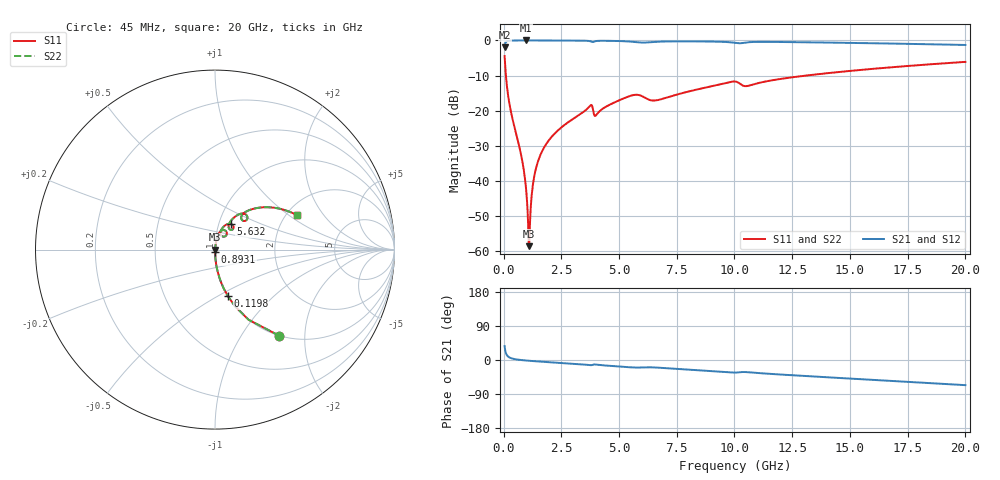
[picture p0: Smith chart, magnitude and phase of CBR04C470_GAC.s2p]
! S-parameter model data by Modelithics Inc.  support@modelithics.com 813-866-6335  Tampa FL USA
! S-Parameter data specifications:
! Substrate: 20-mil Rogers 4350B, substrate thickness, H=0.508mm, Dielectric constant, Er=3.75
! PCB Mounting Pad Footprint: Pad width, PadW=0.52mm , Pad length, PadL=0.52mm , Pad gap, PadG (edge-to-edge)=0.28mm , Reference planes=1.32mm apart
#  GHz  S  MA  R 50
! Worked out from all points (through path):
!   801 points, 45 MHz to 20 GHz, reference 50 ohm
!   highest |S21| = -0.01 dB at 967.9 MHz (marker M1); lowest = -1.9 dB at 45 MHz (marker M2)
!   group delay of S21, straight-line fit = 9.44 ps
!   lowest |S11| = -58.6 dB at 1.093 GHz (marker M3), VSWR 1.00, Z = 50.1 - j0.0592 ohm
!   |S11| at or under -10 dB: 100.8 MHz to 13.11 GHz (13.01 GHz wide, 197 % of centre)
!   |S22| runs from -58.6 to -4.4 dB; largest |S21 - S12| = 0
!   S11 on the Smith chart (normalised r, x): 45 MHz: 1.00, -1.50; 119.8 MHz: 1.00, -0.56; 893.1 MHz: 1.00, -0.03; 5.632 GHz: 1.14, +0.33; 20 GHz: 2.27, +1.16
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0.045  0.5995 -53.2  0.8002 36.8  0.8002 36.8  0.5995 -53.2
0.119831  0.2682 -74.6  0.963 15.3  0.963 15.3  0.2682 -74.6
0.319381  0.0964 -84.7  0.9948 4.9  0.9948 4.9  0.0964 -84.7
0.893088  0.01307 -86.8  0.999 -0.9  0.999 -0.9  0.01307 -86.8
0.967919  0.008082 -84.4  0.999 -1.3  0.999 -1.3  0.008082 -84.4
1.017806  0.005021 -80.1  0.999 -1.6  0.999 -1.6  0.005021 -80.1
1.092637  0.001176 -30.2  0.9989 -2.0  0.9989 -2.0  0.001176 -30.2
1.167469  0.003681 70.7  0.9989 -2.3  0.9989 -2.3  0.003681 70.7
1.267244  0.008674 79.8  0.9988 -2.8  0.9988 -2.8  0.008674 79.8
1.367019  0.01341 81.7  0.9987 -3.3  0.9987 -3.3  0.01341 81.7
1.691288  0.02734 82.6  0.9983 -4.7  0.9983 -4.7  0.02734 82.6
2.314881  0.0509 81.0  0.997 -7.2  0.997 -7.2  0.0509 81.0
3.387462  0.09222 76.4  0.9922 -11.5  0.9922 -11.5  0.09222 76.4
3.761619  0.1191 66.3  0.9721 -13.6  0.9721 -13.6  0.1191 66.3
4.011056  0.08637 67.3  0.9806 -12.2  0.9806 -12.2  0.08637 67.3
5.6324  0.1669 58.7  0.9529 -19.7  0.9529 -19.7  0.1669 58.7
6.704981  0.1421 57.1  0.9589 -20.2  0.9589 -20.2  0.1421 57.1
10.0225  0.2599 47.3  0.9232 -33.2  0.9232 -33.2  0.2599 47.3
10.52138  0.2235 48.1  0.9364 -31.9  0.9364 -31.9  0.2235 48.1
13.36496  0.3234 45.4  0.9386 -43.3  0.9386 -43.3  0.3234 45.4
16.68248  0.4117 34.2  0.9041 -54.8  0.9041 -54.8  0.4117 34.2
20  0.4949 22.9  0.8615 -66.4  0.8615 -66.4  0.4949 22.9
